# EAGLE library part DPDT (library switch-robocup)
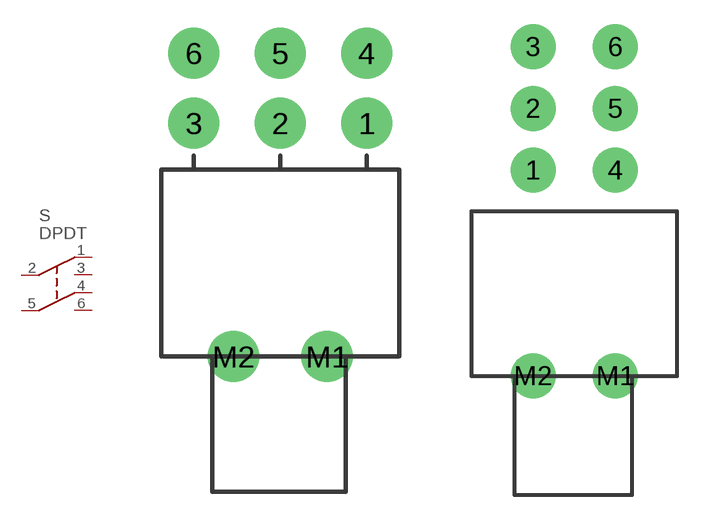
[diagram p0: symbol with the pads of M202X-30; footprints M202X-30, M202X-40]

Designator prefix S

## DPDTM2022-30  [M202X-30]
1  NC1
2  C1
3  NO1
4  NC2
5  C2
6  NO2

## DPDTM2022-40  [M202X-40]
Pads as for M202X-30

## Footprint M202X-30 (pad centres in mm)
drill 1.854: 1 4.699,12.7; 2 0,12.7; 3 -4.699,12.7; 4 4.699,16.51; 5 0,16.51; 6 -4.699,16.51; M1 2.54,0; M2 -2.54,0

## Footprint M202X-40 (pad centres in mm)
drill 1.854: 1 -2.54,12.7; 2 -2.54,16.51; 3 -2.54,20.32; 4 2.54,12.7; 5 2.54,16.51; 6 2.54,20.32; M1 2.54,0; M2 -2.54,0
